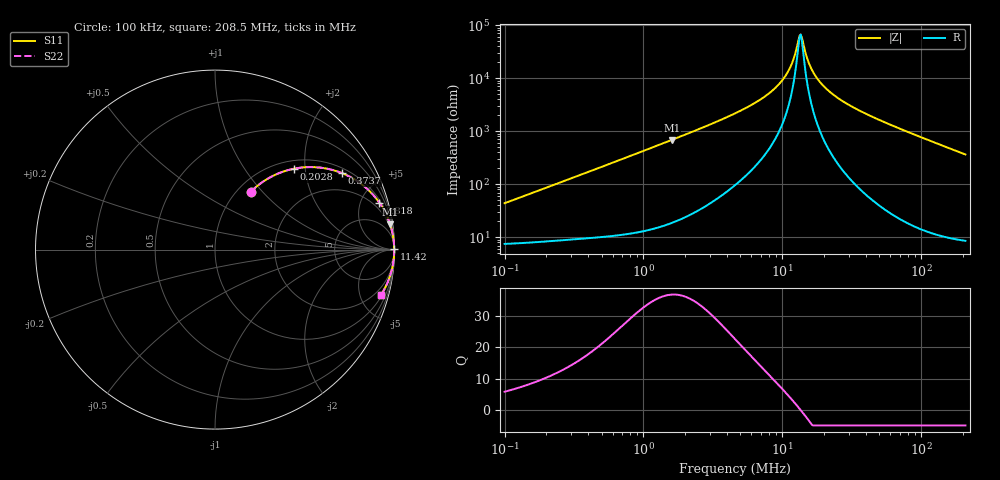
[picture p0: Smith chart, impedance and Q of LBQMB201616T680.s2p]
! LBQMB201616T680  S-PARAMETER MODEL  ( General Type )
! Model Generated by TAIYO YUDEN Corporation (http://www.ty-top.com)
! Version 1.0
! TAIYO YUDEN Control No. 191025NI43SB-FBB
! Copyright(c) 2019 TAIYO YUDEN CO.,LTD. All Rights Reserved.
! Product Description (link to TY-COMPAS)
! https://ds.yuden.co.jp/TYCOMPAS/or/detail?pn=LBQMB201616T680J&u=M
! Products Name : Inductors
! Characteristics :
!  Inductance : 68 uH , SRF(min) : 11 MHz , DC Resistance(max) : 9.1 Ohm , Rated Current : 90 mA
!  Case Size : 2.0 x 1.6 / 0.079 x 0.063 [mm/inch] , Thickness : 1.6 / 0.063 [mm/inch]
!  (Conditions: Temperature = 25 degC , DC Bias Current/Voltage = 0A / 0V)
! External Node Assignments :
!  1  o---GGG---o  2
! GND o---------o GND
! Frequency Range : 0.1MHz  -  208.503118MHz  [ 402 STEP ]
# MHz S RI R 50
! Freq[MHz].  S11 Real  S11 Imag  S21 Real  S21 Imag  S12 Real  S12 Imag  S22 Real  S22 Imag
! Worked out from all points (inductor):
!   401 points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, 100 kHz to 208.5 MHz, reference 50 ohm
!   read as one part in series: L = 68.8 uH near 103.9 kHz
!   highest Q = 36.8 at 1.597 MHz (marker M1), where L = 68.3 uH
!   self-resonance near 13.31 MHz
!   S11 on the Smith chart (normalised r, x): 100 kHz: 1.15, +0.87; 202.8 kHz: 1.17, +1.74; 373.7 kHz: 1.19, +3.19; 818 kHz: 1.24, +6.96; 11.42 MHz: open; 208.5 MHz: 1.17, -7.30
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0.1  0.1997 0.3225  0.8003 -0.3225  0.8003 -0.3225  0.1997 0.3225
0.202777  0.4396 0.4506  0.5604 -0.4506  0.5604 -0.4506  0.4396 0.4506
0.359709  0.6921 0.4321  0.3079 -0.4321  0.3079 -0.4321  0.6921 0.4321
0.37372  0.7073 0.4263  0.2927 -0.4263  0.2927 -0.4263  0.7073 0.4263
0.818005  0.9163 0.2605  0.0837 -0.2605  0.0837 -0.2605  0.9163 0.2605
1.293906  0.9638 0.1733  0.0362 -0.1733  0.0362 -0.1733  0.9638 0.1733
1.596534  0.9755 0.1417  0.0245 -0.1417  0.0245 -0.1417  0.9755 0.1417
4.654297  0.996 0.0446  0.00401 -0.0446  0.00401 -0.0446  0.996 0.0446
8.415604  0.998 0.0173  0.00199 -0.0173  0.00199 -0.0173  0.998 0.0173
9.994598  0.9983 0.0108  0.00173 -0.0108  0.00173 -0.0108  0.9983 0.0108
11.42483  0.9984 0.00595  0.00159 -0.00595  0.00159 -0.00595  0.9984 0.00595
12.09882  0.9985 0.00392  0.00154 -0.00392  0.00154 -0.00392  0.9985 0.00392
13.05973  0.9985 0.00122  0.0015 -0.00122  0.0015 -0.00122  0.9985 0.00122
13.56844  0.9985 -0.000128  0.00148 0.000128  0.00148 0.000128  0.9985 -0.000128
14.09696  0.9985 -0.00148  0.00147 0.00148  0.00147 0.00148  0.9985 -0.00148
15.51009  0.9985 -0.00487  0.00146 0.00487  0.00146 0.00487  0.9985 -0.00487
16.42508  0.9985 -0.00692  0.00147 0.00692  0.00147 0.00692  0.9985 -0.00692
19.50687  0.9984 -0.0133  0.00155 0.0133  0.00155 0.0133  0.9984 -0.0133
25.00684  0.9981 -0.0232  0.00188 0.0232  0.00188 0.0232  0.9981 -0.0232
35.27109  0.9971 -0.0395  0.00292 0.0395  0.00292 0.0395  0.9971 -0.0395
59.08252  0.993 -0.0732  0.00698 0.0732  0.00698 0.0732  0.993 -0.0732
208.5031  0.9251 -0.2517  0.0749 0.2517  0.0749 0.2517  0.9251 -0.2517
